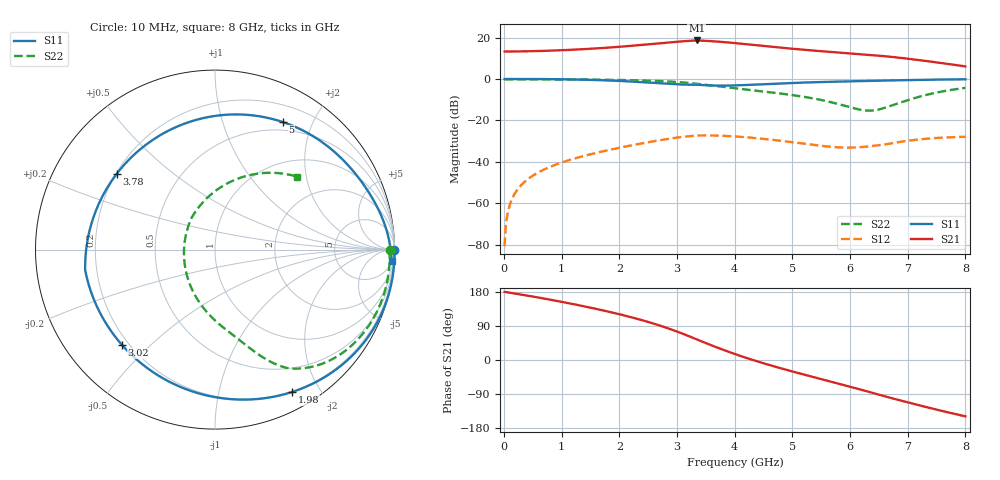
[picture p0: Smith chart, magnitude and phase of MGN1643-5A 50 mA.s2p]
! Port[1] = GATE
! Port[2] = DRAIN
! [Type]  S-parameter s2p file touchstone ver. 1.0
! [Object]  MGN1643-5A
! [Bias]  50 mA
! [Version]  1.0
! [Date]  Thu May 19 10:54:03 2026
! [Source]  This file was created in JSC "ICC Milandr".
! [Disclaimer] Property of JSC "ICC Milandr". Unauthorized reproduction and/or distribution is strictly prohibited.
!  The file and the data are provided "AS IS" and with all faults and disclaim all warranties, express and implied, including
!  without limitation any implied warranties of merchantability, fitness for a particular purpose.
!  JSC "ICC Milandr" assumes no liability for:
!  1) the accuracy of the data provided;
!  2) the proper functioning of this data;
!  3) infringement of patents, copyrights or intellectual property rights resulting from the use of this data.
!  JSC "ICC Milandr" reserves the right to make changes to the products and the data without prior notice.
!  Please, be aware that your receipt and use of the file provided shall serve as acceptance of these terms and conditions.
!  If you do not accept these terms, you should return or destroy this file and any other accompanying information immediately.
# Hz S MA R 12.5
! freq  S11mag  S11ang  S21mag  S21ang  S12mag  S12ang  S22mag  S22ang
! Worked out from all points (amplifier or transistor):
!   800 points, 10 MHz to 8 GHz, reference 12.5 ohm
!   highest |S21| = 18.6 dB at 3.34 GHz (marker M1)
!   |S21| within 3 dB of that: 2.026 GHz to 4.628 GHz (2.602 GHz wide, 78.2 % of centre)
!   unconditionally stable (mu >= 1): 5.374 GHz to 6.166 GHz
!   at 1.34 GHz: K = 0.22, MSG = 25.9 dB, |S12| = -37.4 dB
!   at 4.01 GHz: K = 0.64, MSG = 22.5 dB, |S12| = -27.7 dB
!   at 8 GHz: K = 0.34, MSG = 17.0 dB, |S12| = -27.9 dB
!   S11 on the Smith chart (normalised r, x): 10 MHz: open; 1.98 GHz: 0.20, -1.67; 3.02 GHz: 0.17, -0.41; 3.78 GHz: 0.20, +0.33; 5 GHz: 0.39, +1.59; 8 GHz: 6, -30
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1e7  1 -0.2  4.607 179.7  9.29e-05 86.6  0.9729 -0.1
1.1e8  1.001 -2.8  4.61 177.3  0.001013 87.5  0.9737 -1.5
3.1e8  1.001 -7.8  4.643 172.3  0.002869 83.9  0.975 -4.1
1.35e9  0.9671 -37.3  5.224 142.9  0.01355 61.1  0.9693 -18.8
1.98e9  0.9024 -61.5  5.961 121.5  0.02168 43.9  0.9491 -29.0
2.35e9  0.8468 -80.7  6.579 106.9  0.02738 31.7  0.9267 -35.9
2.68e9  0.7907 -103.3  7.249 92.0  0.03305 18.7  0.8951 -42.9
3.02e9  0.7419 -134.4  7.982 74.0  0.03894 2.7  0.8433 -51.0
3.19e9  0.7305 -153.2  8.302 63.9  0.0415 -6.5  0.8075 -55.2
3.34e9  0.7323 -171.1  8.517 54.4  0.04325 -15.2  0.7703 -58.9
3.56e9  0.7006 165.1  8.245 40.9  0.04354 -26.7  0.7086 -62.9
3.78e9  0.6915 142.4  7.842 28.0  0.04278 -37.2  0.6502 -66.4
4.01e9  0.7013 121.2  7.347 15.4  0.04114 -46.7  0.5957 -69.7
4.25e9  0.7238 102.4  6.812 3.2  0.03881 -55.0  0.5457 -73.0
4.49e9  0.7508 86.9  6.302 -8.2  0.03612 -61.5  0.5008 -76.8
4.74e9  0.7786 73.5  5.82 -19.3  0.03311 -66.4  0.4563 -81.5
5e9  0.8047 62.1  5.379 -30.3  0.02993 -69.0  0.4097 -87.7
5.34e9  0.8338 49.8  4.889 -44.1  0.02603 -68.4  0.3447 -98.6
6e9  0.8794 31.8  4.142 -70.5  0.02217 -52.3  0.2085 -139.6
6.67e9  0.9228 17.9  3.482 -98.7  0.02733 -35.4  0.2185 127.2
7.3e9  0.9586 7.5  2.745 -123.4  0.03602 -47.6  0.4065 73.7
8e9  0.9862 -3.7  2.012 -148.7  0.04036 -65.0  0.6127 41.6
